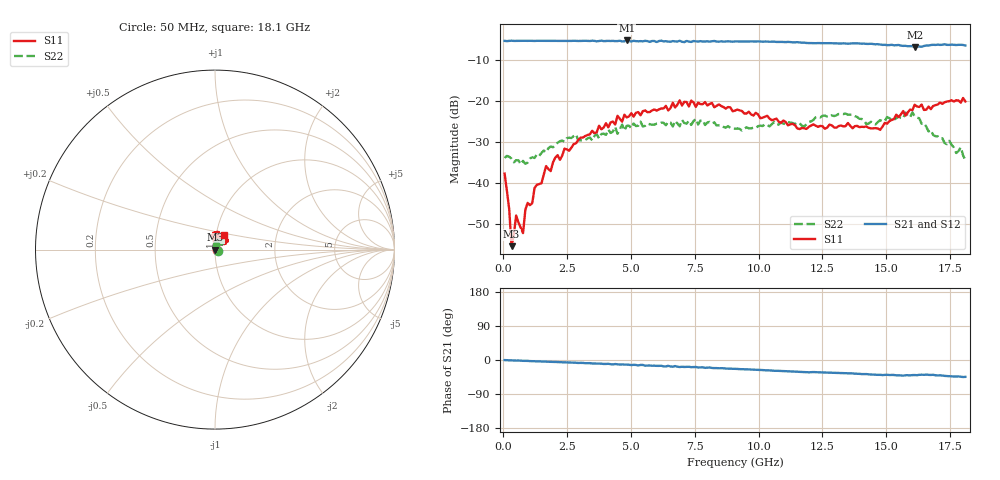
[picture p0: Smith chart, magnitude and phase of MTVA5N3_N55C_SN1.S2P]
! Network Analyzer HP8720D.06.14 Serial No. US36140669
! 11 May 2005  11:30:21
! Frequency  S11  S21  S12  S22
# HZ  S  DB R 50
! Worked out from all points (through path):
!   201 points, 50 MHz to 18.1 GHz, reference 50 ohm
!   highest |S21| = -5.29 dB at 4.833 GHz (marker M1); lowest = -6.9 dB at 16.11 GHz (marker M2)
!   group delay of S21, straight-line fit = 6.99 ps
!   lowest |S11| = -55.5 dB at 320.8 MHz (marker M3), VSWR 1.00, Z = 50.2 - j0.0378 ohm
!   |S11| at or under -10 dB: start of sweep to end of sweep
!   |S22| runs from -35.5 to -22.8 dB; largest |S21 - S12| = 0.018
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5e7  -37.80 -17.5  -5.40 -0.2  -5.44 -0.7  -33.95 -19.4
2.305e8  -46.50 -1.1  -5.40 -0.7  -5.37 -1.2  -33.68 -5.5
3.2075e8  -55.50 -13.0  -5.35 -0.7  -5.38 -1.0  -34.14 -2.9
5.0125e8  -48.04 -20.1  -5.39 -1.5  -5.37 -1.8  -34.52 6.3
7.72e8  -52.32 28.2  -5.39 -2.2  -5.37 -2.4  -34.69 13.8
9.525e8  -44.94 34.3  -5.39 -2.3  -5.37 -2.9  -35.11 21.8
1.133e9  -44.99 35.0  -5.38 -3.1  -5.42 -3.5  -33.82 35.1
1.22325e9  -41.29 38.8  -5.41 -3.2  -5.40 -3.7  -33.97 33.1
1.6745e9  -35.95 52.7  -5.39 -4.3  -5.40 -4.7  -32.59 49.5
1.855e9  -37.17 54.1  -5.41 -4.8  -5.40 -5.2  -31.17 56.1
2.12575e9  -33.29 61.4  -5.39 -5.5  -5.40 -5.8  -30.26 60.8
3.1185e9  -28.99 62.3  -5.39 -7.7  -5.42 -8.3  -29.72 88.7
4.83325e9  -24.08 75.4  -5.29 -12.2  -5.39 -13.2  -26.13 78.7
6.09675e9  -22.12 78.2  -5.44 -15.5  -5.39 -16.0  -25.56 78.7
6.909e9  -19.93 82.6  -5.37 -18.6  -5.48 -18.3  -26.24 67.4
9.075e9  -22.42 98.4  -5.53 -23.4  -5.50 -23.9  -26.85 54.6
1.21435e10  -25.78 92.2  -5.95 -31.8  -5.92 -32.4  -24.70 55.2
1.512175e10  -24.99 34.9  -6.43 -39.6  -6.32 -39.8  -24.26 59.8
1.61145e10  -20.99 37.9  -6.85 -39.7  -6.66 -40.4  -23.85 48.7
1.7739e10  -19.89 57.5  -6.41 -43.6  -6.48 -43.8  -32.76 75.8
1.79195e10  -20.47 59.6  -6.34 -44.3  -6.20 -44.1  -31.35 80.5
1.81e10  -20.19 58.6  -6.53 -44.5  -6.52 -45.8  -34.51 70.1
